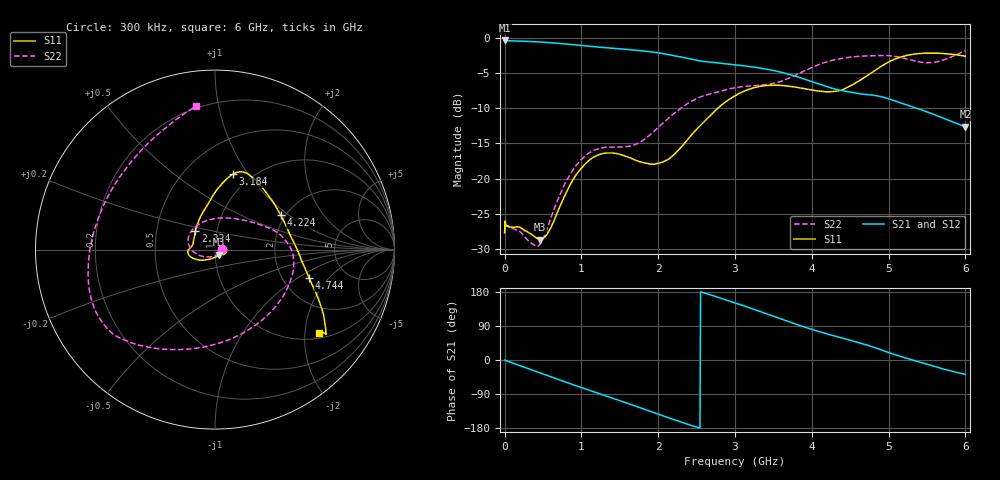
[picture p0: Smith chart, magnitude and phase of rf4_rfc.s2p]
!Agilent Technologies,M9375A,MY55441453,A.02.50.04
!Agilent M9375A: A.02.50.04
!Date: Monday, December 12, 2016 11:30:03
!Correction: S11(Full 2 Port(1,2))
!S21(Full 2 Port(1,2))
!S12(Full 2 Port(1,2))
!S22(Full 2 Port(1,2))
!S2P File: Measurements: S11, S21, S12, S22:
# Hz S  dB  R 50
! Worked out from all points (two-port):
!   751 points, 300 kHz to 6 GHz, reference 50 ohm
!   highest |S21| = -0.37 dB at 8.3 MHz (marker M1); lowest = -12.6 dB at 6 GHz (marker M2)
!   |S21| within 3 dB of the highest: start of sweep to 2.608 GHz
!   lowest |S11| = -28.7 dB at 456.3 MHz (marker M3), VSWR 1.08, Z = 52.4 - j2.95 ohm
!   |S11| at or under -10 dB: start of sweep to 2.776 GHz
!   |S22| runs from -29.6 to -1.8 dB; largest |S21 - S12| = 0.0012
!   S11 on the Smith chart (normalised r, x): 300 kHz: 1.09, -0.00; 2.224 GHz: 0.79, +0.17; 3.184 GHz: 0.82, +0.85; 4.224 GHz: 1.89, +0.87; 4.744 GHz: 2.78, -1.27; 6 GHz: 1.15, -2.36
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300000  -27.70 -2.2  -0.39 -0.1  -0.39 -0.1  -27.78 1.0
8299600  -26.01 3.3  -0.37 -0.6  -0.37 -0.6  -26.04 2.5
4.562772e8  -28.66 -49.7  -0.59 -33.8  -0.59 -33.8  -29.43 -84.1
5.842708e8  -27.31 -89.2  -0.68 -43.2  -0.68 -43.2  -26.15 -124.4
7.762612e8  -22.60 -129.9  -0.86 -57.0  -0.85 -57.0  -20.92 -158.2
1.00025e9  -18.50 -152.9  -1.10 -72.8  -1.10 -72.8  -17.26 177.0
1.232238e9  -16.58 -167.6  -1.33 -88.8  -1.33 -88.8  -15.72 153.5
1.496225e9  -16.54 -178.9  -1.56 -106.9  -1.56 -107.0  -15.51 119.6
2.0002e9  -17.83 159.6  -2.14 -142.9  -2.14 -142.9  -12.74 45.3
2.224189e9  -16.39 136.0  -2.56 -158.7  -2.56 -158.7  -10.60 27.1
2.632168e9  -11.52 97.3  -3.41 175.0  -3.41 174.9  -8.11 8.1
3.00015e9  -8.23 82.0  -3.84 150.9  -3.83 150.8  -7.09 -7.4
3.184141e9  -7.31 76.8  -4.07 138.2  -4.07 138.1  -6.85 -21.6
3.40813e9  -6.78 71.0  -4.45 122.2  -4.45 122.1  -6.66 -46.5
3.648118e9  -6.81 64.3  -5.02 104.8  -5.02 104.7  -5.98 -78.4
4.0001e9  -7.42 47.0  -6.21 80.8  -6.21 80.7  -4.21 -115.5
4.224089e9  -7.67 27.5  -7.03 67.4  -7.03 67.3  -3.32 -128.9
4.744063e9  -5.22 -16.9  -8.09 37.8  -8.09 37.8  -2.56 -144.4
5.00005e9  -3.43 -28.4  -8.66 19.8  -8.65 19.7  -2.54 -154.8
5.416029e9  -2.22 -37.0  -10.19 -6.4  -10.19 -6.5  -3.45 164.3
5.720014e9  -2.24 -37.3  -11.44 -24.2  -11.44 -24.3  -3.11 122.8
6e9  -2.61 -38.7  -12.64 -37.9  -12.64 -37.9  -1.85 97.4
